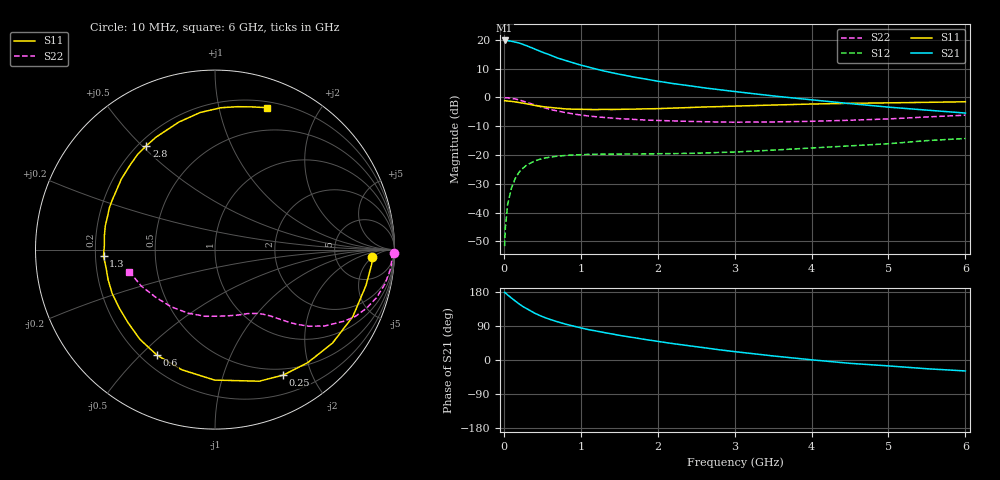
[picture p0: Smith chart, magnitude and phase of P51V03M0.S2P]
! SIEMENS Small Signal Semiconductors
! BFP183
! Si NPN RF Bipolar Junction Transistor in SOT143
! VCE = 1 V  IC = 3 mA
! Common Emitter S-Parameters:  March  1996
# GHz  S  MA  R  50
!  f  S11  S21  S12  S22
! GHz  MAG  ANG  MAG  ANG  MAG  ANG  MAG  ANG
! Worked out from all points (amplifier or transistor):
!   36 points, 10 MHz to 6 GHz, reference 50 ohm
!   highest |S21| = 19.8 dB at 10 MHz (marker M1)
!   |S21| within 3 dB of that: start of sweep to 404.5 MHz
!   unconditionally stable (mu >= 1): 1.792 GHz to end of sweep
!   at 250 MHz: K = 0.16, MSG = 21.5 dB, |S12| = -24.6 dB
!   at 1.4 GHz: K = 0.82, MSG = 14.2 dB, |S12| = -19.7 dB
!   at 6 GHz: K = 1.05, MAG = 3.1 dB, |S12| = -14.3 dB
!   S11 on the Smith chart (normalised r, x): 10 MHz: 14, -5; 250 MHz: 0.42, -1.60; 600 MHz: 0.26, -0.56; 1.3 GHz: 0.23, -0.03; 2.8 GHz: 0.23, +0.52; 6 GHz: 0.26, +1.40
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0.01  0.8784 -2.6  9.791 178.6  0.0026 88.7  0.9962 -1.1
0.02  0.8767 -5.4  9.716 177.2  0.0055 87.5  0.9862 -2.3
0.05  0.8647 -13.3  9.709 171.6  0.014 84.5  0.9862 -5.7
0.1  0.8539 -25.9  9.482 163.4  0.0268 75.3  0.9663 -11.4
0.15  0.8366 -38.5  9.142 155.4  0.0395 69.0  0.939 -16.6
0.2  0.8147 -50.6  8.844 147.8  0.0505 63.5  0.9039 -21.3
0.25  0.7958 -61.5  8.357 140.8  0.0591 57.5  0.8638 -25.7
0.3  0.7736 -71.4  7.888 135.2  0.0672 52.9  0.8211 -29.1
0.4  0.727 -90.2  6.972 123.7  0.0788 44.7  0.7452 -34.8
0.5  0.6945 -105.5  6.133 114.5  0.0868 38.0  0.6773 -39.1
0.6  0.671 -118.8  5.485 107.1  0.0918 33.1  0.6222 -42.1
0.7  0.6519 -129.9  4.844 100.7  0.0956 29.5  0.5796 -44.4
0.8  0.633 -139.9  4.403 94.8  0.0981 26.4  0.5463 -46.1
1.1  0.6187 -164.3  3.375 80.2  0.1024 20.5  0.4761 -50.6
1.3  0.6222 -176.6  2.889 72.6  0.1033 18.0  0.449 -53.3
1.7  0.6265 162.9  2.25 58.7  0.1043 15.8  0.4151 -59.1
2.2  0.6533 143.0  1.743 43.2  0.1057 15.7  0.3916 -67.7
2.8  0.6937 123.4  1.366 27.0  0.1107 17.8  0.3744 -80.6
3.5  0.7385 105.8  1.064 10.7  0.1215 19.5  0.3754 -98.2
4.5  0.7911 87.6  0.782 -8.8  0.1441 19.6  0.4017 -127.7
5.5  0.8223 75.2  0.602 -23.1  0.1778 17.1  0.4583 -153.7
6  0.8417 69.9  0.536 -28.9  0.1935 13.6  0.4923 -165.5
